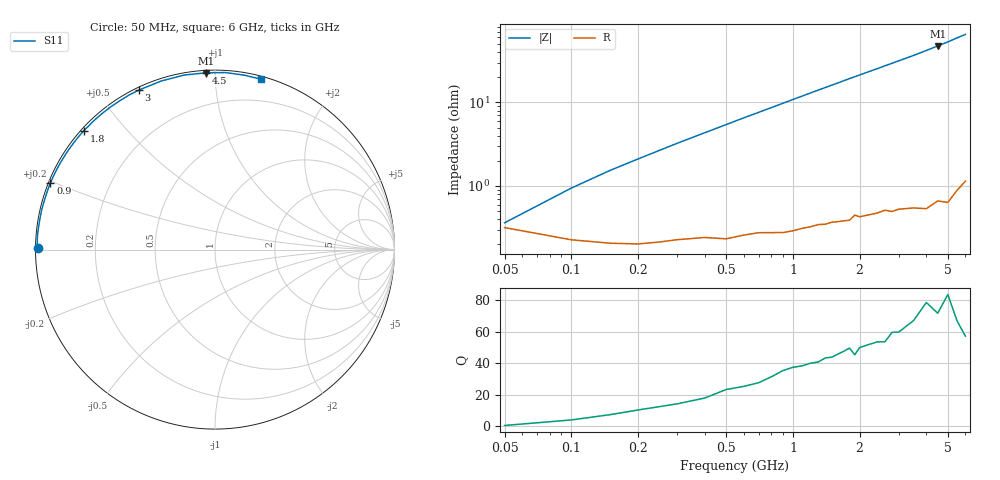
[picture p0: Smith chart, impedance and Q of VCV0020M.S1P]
! Infineon Technologies  Discrete & RF Semiconductors
! BBY 56-03
! Si Tuning Diode in SOD323
! VR =
! S-Parameters:  June  1999
# GHz  S  MA  R  50
!  f  S11
! GHz  MAG  ANG
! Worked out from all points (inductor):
!   34 points, 50 MHz to 6 GHz, reference 50 ohm
!   read as one part to ground: L = 1.62 nH near 100 MHz
!   highest Q = 78.4 at 4.5 GHz (marker M1), where L = 1.68 nH
!   S11 on the Smith chart (normalised r, x): 50 MHz: 0.01, +0.00; 900 MHz: 0.01, +0.20; 1.8 GHz: 0.01, +0.39; 3 GHz: 0.01, +0.63; 4.5 GHz: 0.01, +0.95; 6 GHz: 0.02, +1.30
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0.05  0.9874 179.6
0.1  0.991 177.9
0.15  0.9918 176.5
0.25  0.9915 173.9
0.4  0.9905 170.1
0.5  0.9908 167.6
0.6  0.9899 165.1
0.8  0.9893 160.3
0.9  0.9894 157.9
1  0.989 155.5
1.1  0.9883 153.2
1.3  0.9873 148.6
1.5  0.9867 144.2
1.6  0.9867 142.1
1.7  0.9866 139.9
1.8  0.9865 137.8
2  0.9856 133.8
2.2  0.9853 129.9
2.4  0.985 126.2
2.6  0.9844 122.5
2.8  0.9854 119.0
3  0.985 115.6
3.5  0.9859 107.7
4  0.9875 100.0
4.5  0.9861 93.0
5  0.9881 86.6
5.5  0.9854 80.3
6  0.9832 75.0
